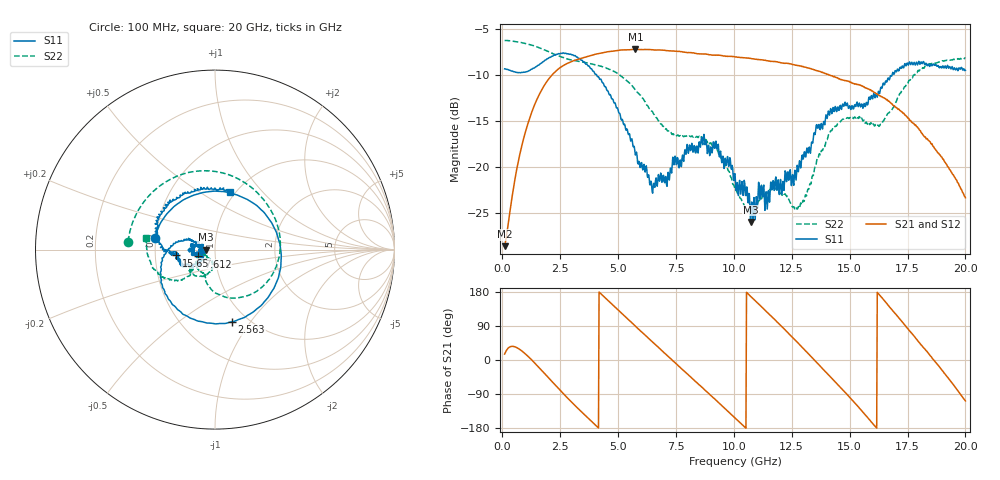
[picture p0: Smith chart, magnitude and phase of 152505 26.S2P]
!  2-Port S-parameters saved by WinCal
! VAR MeasName=S-Parameters (CALIBRATED_DATA) read from VNA (N5230C)
! VAR MeasDate=4/10/2015 9:30:56 AM
! VAR NAME=152505 26
! VAR FILENAME=152505 26.S2P
! VAR DATE=4/10/2015 9:30:56 AM
! VAR PHYS_PORTS=1,2
# Hz S DB R 50
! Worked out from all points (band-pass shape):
!   801 points, 100 MHz to 20 GHz, reference 50 ohm
!   highest |S21| = -7.23 dB at 5.747 GHz (marker M1); lowest = -28.7 dB at 100 MHz (marker M2)
!   |S21| within 3 dB of the highest: 2.078 GHz to 14.36 GHz (12.28 GHz wide, 149 % of centre)
!   lowest |S11| = -26.0 dB at 10.72 GHz (marker M3), VSWR 1.11, Z = 45.2 - j0.0922 ohm
!   |S11| at or under -10 dB: 4.066 GHz to 16.83 GHz (12.77 GHz wide, 122 % of centre)
!   |S22| runs from -24.7 to -6.3 dB; largest |S21 - S12| = 0.0066
!   S11 on the Smith chart (normalised r, x): 100 MHz: 0.50, +0.07; 2.563 GHz: 0.85, -0.82; 7.612 GHz: 0.83, -0.06; 15.65 GHz: 0.64, -0.04; 20 GHz: 0.94, +0.68
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1e8  -9.36 168.9  -28.65 15.6  -28.61 15.7  -6.27 174.7
8.71125e8  -9.75 86.6  -17.43 22.5  -17.43 22.5  -6.53 134.4
1.617375e9  -8.86 7.2  -12.05 -21.7  -12.04 -21.8  -7.09 96.5
2.04025e9  -8.11 -33.3  -10.35 -49.7  -10.35 -49.8  -7.53 76.2
2.562625e9  -7.68 -76.8  -9.12 -84.1  -9.11 -84.2  -8.07 53.0
3.43325e9  -8.42 -132.9  -8.20 -137.5  -8.20 -137.5  -8.61 16.1
4.502875e9  -11.60 -178.8  -7.53 160.6  -7.56 160.4  -9.30 -29.8
5.746625e9  -18.74 159.5  -7.23 89.3  -7.29 89.3  -11.65 -80.7
6.741625e9  -20.86 -179.0  -7.31 33.3  -7.31 33.0  -15.02 -107.5
7.61225e9  -19.99 -157.5  -7.45 -15.9  -7.50 -15.9  -16.63 -114.7
8.831125e9  -17.71 -174.8  -7.77 -84.0  -7.82 -84.1  -17.23 -138.2
1.005e10  -20.77 167.4  -8.05 -152.9  -8.07 -153.0  -22.49 -157.2
1.072162e10  -26.01 -178.8  -8.22 167.9  -8.26 168.2  -24.49 -140.5
1.206488e10  -23.03 -153.0  -8.71 88.4  -8.70 88.7  -23.06 -135.5
1.27365e10  -19.85 -146.5  -8.98 47.0  -8.93 46.9  -24.63 -123.5
1.338325e10  -17.35 -140.6  -9.41 6.1  -9.36 6.2  -21.05 -99.3
1.457725e10  -13.42 -165.4  -10.48 -71.1  -10.38 -71.1  -15.13 -122.7
1.564688e10  -13.17 -171.4  -11.38 -143.0  -11.45 -142.7  -15.09 -140.5
1.669162e10  -10.52 177.8  -12.88 142.7  -12.93 141.5  -14.16 -134.2
1.738812e10  -8.79 156.7  -14.40 91.9  -14.41 91.2  -11.29 -140.2
1.825875e10  -8.89 130.7  -16.74 28.6  -16.83 28.1  -9.07 -159.5
2e10  -9.53 75.9  -23.38 -107.9  -23.44 -107.3  -8.20 170.7
